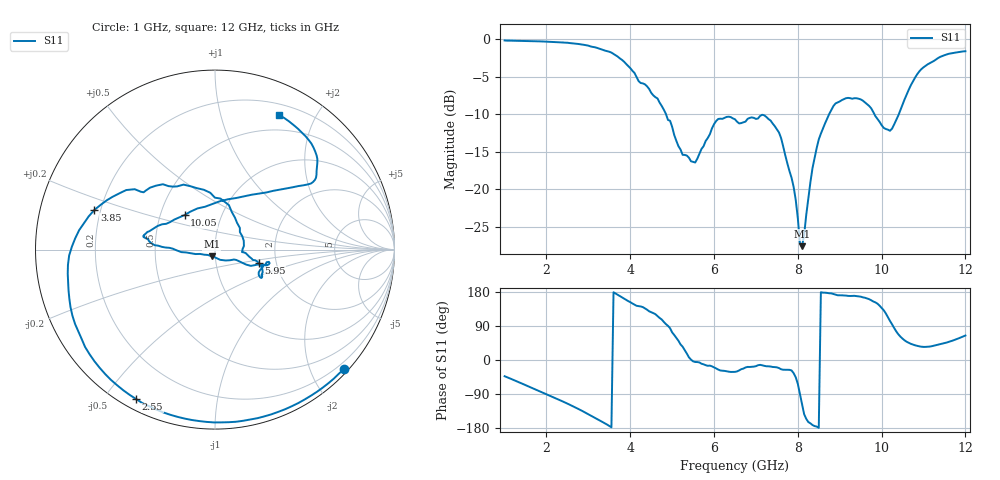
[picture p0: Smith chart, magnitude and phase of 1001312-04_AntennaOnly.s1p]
! 1/26/2023 7:01:49 AM
! D:\1001312-04WITHOUTMATCHING.S1P
! CHANNEL.1
! TR.MEASUREMENT
! CORRECTED.DATA
! RF.CORRECTION: ONE.PORT.CAL.PORT[1]
! AVERAGING.OFF
! IF.BANDWIDTH: 1KHZ
! SWEEPTYPE:  FREQ.SWEEP(Linear)
! Reference Plane Port Info
! PORT:  PORT1
! DISTANCE:  4.1659 cm
! TIME:  139.0043 ps
! PHASE.OFFSET:  0 °
! LOSS:  0  dB
! REF.LOSS:  0  dB
! REF.FREQ:  1 GHz
! Power Info
! POWER:  -10  dBm
! EFF.POWER:  -10  dBm
! SOURCE.ATTEN:  0  dB
! TEST.ATTEN:  0  dB
# GHZ S RI R 50.0
! FREQ.GHZ  S11RE  S11IM
!; PortSelection: Port_1
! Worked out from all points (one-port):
!   221 points, 1 GHz to 12 GHz, reference 50 ohm
!   lowest |S11| = -27.6 dB at 8.1 GHz (marker M1), VSWR 1.09, Z = 48.1 - j3.62 ohm
!   |S11| at or under -10 dB: 4.853 GHz to 8.747 GHz (3.895 GHz wide, 57.3 % of centre); 9.827 GHz to 10.41 GHz (583.4 MHz wide, 5.77 % of centre)
!   S11 on the Smith chart (normalised r, x): 1 GHz: 0.08, -2.55; 2.55 GHz: 0.04, -0.60; 3.85 GHz: 0.18, +0.15; 5.95 GHz: 1.62, -0.25; 10.05 GHz: 0.67, +0.27; 12 GHz: 0.32, +1.54
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1  0.7187 -0.6657
1.7  0.236 -0.9394
2.4  -0.3248 -0.892
2.55  -0.4386 -0.8331
3.2  -0.7946 -0.3676
3.75  -0.73 0.1467
3.85  -0.6728 0.2204
4.65  -0.1755 0.3621
5.15  0.1226 0.1497
5.55  0.1501 -0.0137
5.95  0.2436 -0.0731
6.5  0.2497 -0.1518
7.35  0.2738 -0.0848
7.6  0.1997 -0.0906
7.9  0.0851 -0.0591
8.05  0.000608 -0.0437
8.1  -0.0182 -0.0376
8.35  -0.1368 -0.02
8.5  -0.2146 -0.00377
8.85  -0.3567 0.0364
9.25  -0.3968 0.0776
9.7  -0.339 0.1193
10.05  -0.1692 0.1926
10.25  -0.0179 0.2528
10.65  0.3254 0.3276
11  0.5342 0.368
11.35  0.5703 0.4848
12  0.3565 0.7497
